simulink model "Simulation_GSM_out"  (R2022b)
settings: Solver=ode15s  StartTime=0.0  StopTime=15  MaxStep=1e-2  RelTol=1e-7  AbsTol=1e-5  EnableMultiTasking=on
undefined symbols (not defined in the file or in its folder): A, B, C, Contents, D, deconv, parGSM, x0

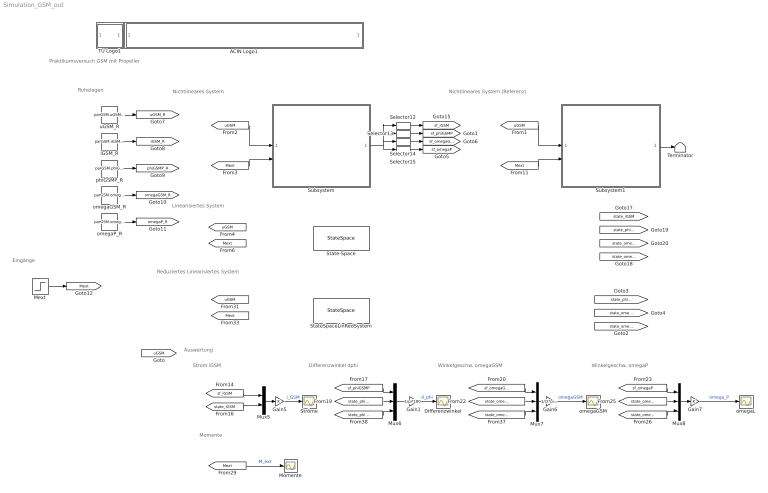
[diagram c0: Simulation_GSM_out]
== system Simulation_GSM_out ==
  note: Eingänge
  note: Ruhelagen
  note: Auswertung
  note: Nichtlineares System
  note: Linearisiertes System
  note: Reduziertes Linearisiertes System
  note: Differenzwinkel dphi
  note: Winkelgeschw. omegaGSM
  note: Winkelgeschw. omegaP
  note: Momente
  note: Praktikumsversuch GSM mit Propeller
  note: Strom iGSM
  note: Nichtlineares System (Referenz)
  ACIN Logo1 : Subsystem
      mask init:
      | s = get_param(gcb,'UserData');
  Differenzwinkel : Scope
  Gain1 : Gain  Gain=1/pi*180
  Gain5 : Gain
  Gain6 : Gain  Gain=1/(2*pi)*60
  Gain7 : Gain
  Mext : Step  Time=11  After=0.25  SampleTime=0
  Momente : Scope
  Mux5 : Mux  Inputs=2
  Mux6 : Mux  Inputs=3
  Mux7 : Mux  Inputs=3
  Mux8 : Mux  Inputs=3
  Selector12 : Selector  InputPortWidth=4  IndexOptions=Index vector (dialog)  Indices=[1]  OutputSizes=1
  Selector13 : Selector  InputPortWidth=4  IndexOptions=Index vector (dialog)  Indices=[2]  OutputSizes=1
  Selector14 : Selector  InputPortWidth=4  IndexOptions=Index vector (dialog)  Indices=[3]  OutputSizes=1
  Selector15 : Selector  InputPortWidth=4  IndexOptions=Index vector (dialog)  Indices=[4]  OutputSizes=1
  State-Space : StateSpace  A=A  B=B  C=C  D=D  InitialCondition=x0
  StateSpaceLinRedSystem : StateSpace  A=A  B=B  C=Contents  D=deconv  InitialCondition=x0
  Ströme : Scope
  Subsystem : Subsystem
  Subsystem1 : Subsystem  mask{iGSM_0=parGSM.iGSM_R, phiGSMP_0=parGSM.phiGSMP_R, omegaGSM_0=parGSM.omegaGSM_R, omegaP_0=parGSM.omegaP_R}
      mask prompts: iGSM_0 "Anfangsbedingung iGSM"; phiGSMP_0 "Anfangsbedingung phiGSMP"; omegaGSM_0 "Anfangsbedingung omegaGSM"; omegaP_0 "Anfangsbedingung omegaP"
  TU Logo1 : Subsystem
      mask init:
      | s = get_param(gcb,'UserData');
  Terminator : Terminator
  iGSM_R : Constant  Value=parGSM.iGSM_R
  omegaGSM : Scope
  omegaGSM_R : Constant  Value=parGSM.omegaGSM_R
  omegaL : Scope
  omegaP_R : Constant  Value=parGSM.omegaP_R
  phiGSMP_R : Constant  Value=parGSM.phiGSMP_R
  uGSM_R : Constant  Value=parGSM.uGSM_R
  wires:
  [Mext] -> Momente/1  "M_ext"
  Mux5/1 -> Gain5/1
  Gain5/1 -> Ströme/1  "i_GSM"
  [sf_iGSM] -> Mux5/1
  Mux6/1 -> Gain1/1
  Gain1/1 -> Differenzwinkel/1  "d_phi"
  [sf_phiGSMP] -> Mux6/1
  Mux7/1 -> Gain6/1
  Gain6/1 -> omegaGSM/1  "omegaGSM"
  Mux8/1 -> Gain7/1
  Gain7/1 -> omegaL/1  "omega_P"
  [sf_omegaP] -> Mux8/1
  [state_phiGSMP] -> Mux6/2
  [state_phiGSMPred] -> Mux6/3
  [state_omegaP] -> Mux8/2
  [state_omegaPred] -> Mux8/3
  [state_iGSM] -> Mux5/2
  [sf_omegaGSM] -> Mux7/1
  [state_omegaGSM] -> Mux7/2
  [state_omegaGSMred] -> Mux7/3
  [uGSM] -> Subsystem/1(uGSM)
  [Mext] -> Subsystem/2(Mext)
  Subsystem/1(y) -> Selector12/1, Selector13/1, Selector14/1, Selector15/1
  Selector13/1 -> [sf_phiGSMP]
  Selector15/1 -> [sf_omegaP]
  Selector12/1 -> [sf_iGSM]
  Selector14/1 -> [sf_omegaGSM]
  omegaGSM_R/1 -> [omegaGSM_R]
  omegaP_R/1 -> [omegaP_R]
  phiGSMP_R/1 -> [phiGSMP_R]
  iGSM_R/1 -> [iGSM_R]
  uGSM_R/1 -> [uGSM_R]
  Mext/1 -> [Mext]
  [uGSM] -> Subsystem1/1(uGSM)
  [Mext] -> Subsystem1/2(Mext)
  Subsystem1/1(y) -> Terminator/1

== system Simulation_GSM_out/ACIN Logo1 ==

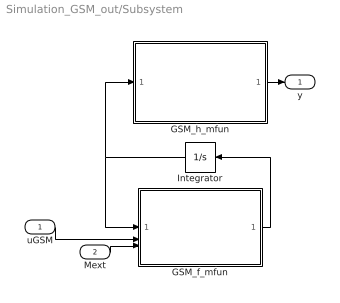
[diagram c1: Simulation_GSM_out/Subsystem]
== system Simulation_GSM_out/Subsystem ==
  uGSM : Inport
  Mext : Inport  Port=2
  GSM_f_mfun : MATLAB Function  TreatAsAtomicUnit=on
  GSM_h_mfun : MATLAB Function  TreatAsAtomicUnit=on
  Integrator : Integrator  InitialCondition=[parGSM.iGSM_R;parGSM.phiGSMP_R;parGSM.omegaGSM_R;parGSM.omegaP_R]
  y : Outport
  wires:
  GSM_f_mfun/1(dx) -> Integrator/1
  uGSM/1 -> GSM_f_mfun/2(u1)
  GSM_h_mfun/1(y) -> y/1
  Integrator/1 -> GSM_f_mfun/1(x), GSM_h_mfun/1(x)
  Mext/1 -> GSM_f_mfun/3(u2)

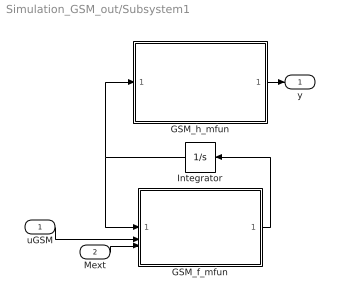
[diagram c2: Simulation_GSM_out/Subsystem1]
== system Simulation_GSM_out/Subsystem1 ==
  uGSM : Inport
  Mext : Inport  Port=2
  GSM_f_mfun : MATLAB Function  TreatAsAtomicUnit=on
  GSM_h_mfun : MATLAB Function  TreatAsAtomicUnit=on
  Integrator : Integrator  InitialCondition=[iGSM_0; phiGSMP_0; omegaGSM_0; omegaP_0]
  y : Outport
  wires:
  GSM_f_mfun/1(dx) -> Integrator/1
  uGSM/1 -> GSM_f_mfun/2(u1)
  GSM_h_mfun/1(y) -> y/1
  Integrator/1 -> GSM_f_mfun/1(x), GSM_h_mfun/1(x)
  Mext/1 -> GSM_f_mfun/3(u2)

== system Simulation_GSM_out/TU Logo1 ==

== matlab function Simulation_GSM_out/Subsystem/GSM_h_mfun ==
function y = GSM_h_mfun(x,parGSM)
%To DO
return;

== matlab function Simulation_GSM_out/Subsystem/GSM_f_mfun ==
function dx = GSM_f_mfun(x,u1,u2,parGSM)
%To Do
return;

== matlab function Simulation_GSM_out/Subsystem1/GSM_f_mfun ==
function dx = GSM_f_mfun(x,u1,u2)
%#codegen
coder.allowpcode('plain');
    dx = GSM_f_mfun(x,u1,u2);
return;

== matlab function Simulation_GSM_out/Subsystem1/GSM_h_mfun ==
function y = GSM_h_mfun(x)
%#codegen
coder.allowpcode('plain');
    y = GSM_h_mfun(x);
return;
